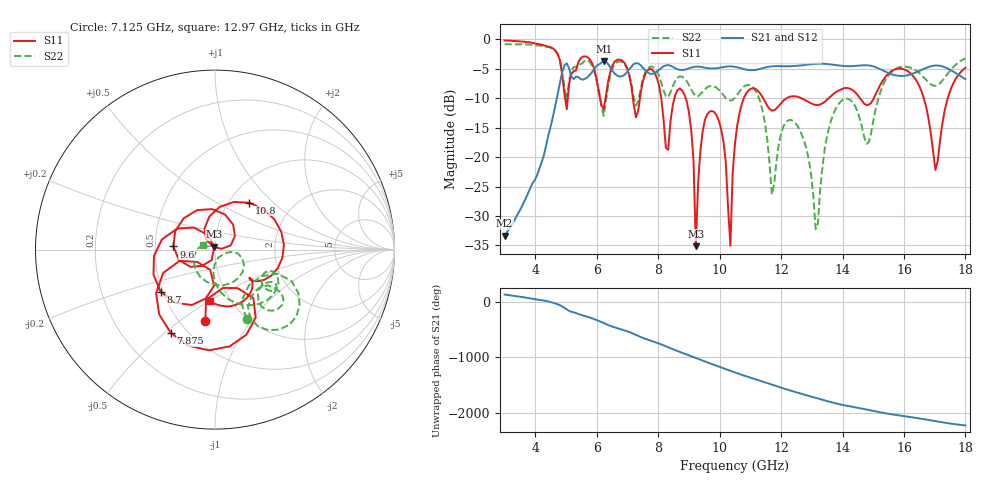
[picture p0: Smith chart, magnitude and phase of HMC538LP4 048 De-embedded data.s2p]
! Chelmsford, MA 01824
! http://www.hittite.com
! Tel: 978-250-3343
! Fax: 978-250-3373
! Device  :  HMC538LP4
! Description:  600 Analog Phase Shifter
! Frequency  :  6.0 GHz - 15.0 GHz
! Package  :  LP4  - 4x4 mm Quad Flatpack No-Lead (QFN) Plastic Package: 24 pin
! Ports  :  2 RF, 1 DC
!  Pin  3  = Rfin  = Port 1
!  Pin  16  = Rfout = Port 2
!  pin  21  = vCTL
! Voltages:  VCTL  = 0 to 5.0 Volts
! Currents :  Vb(V)  Vd(V)  Ib(mA)  Id(mA)
!  0.00  4.80  0.000000	0.483526
! Data:  The device was measured on evaluation board 111296-1.
!  Data was collected using a calibrated network analyzer.
!  The evaluation circuit board was modeled and simulated.This was use
!  to removed the evaluation board circuit from the measured data.
!  The reference plane is the center of the package pin.
! Misc:  Lot #
!Date Measured:  03 - 11 -2009
! Date:  03 - 17 -2009
! Note:
!  Hittite Microwave supplies this data as a sample of measured data at the
!  package pin for this package product.  Your particular data for this product
!  may vary.
!  Data was taken at 25 degrees C.
!  Hittite Microwave reserves the right to change this data at anytime.
# MHz S MA R 50
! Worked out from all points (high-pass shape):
!   201 points, 3 GHz to 18 GHz, reference 50 ohm
!   highest |S21| = -3.68 dB at 6.225 GHz (marker M1); lowest = -33.4 dB at 3 GHz (marker M2)
!   |S21| within 3 dB of the highest: 4.829 GHz to 5.239 GHz (410 MHz wide, 8.14 % of centre); 5.619 GHz to 17.98 GHz (12.36 GHz wide, 105 % of centre)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
!   lowest |S11| = -35.1 dB at 9.225 GHz (marker M3), VSWR 1.04, Z = 49.5 + j1.68 ohm
!   |S11| at or under -10 dB: 8.896 GHz to 10.79 GHz (1.891 GHz wide, 19.2 % of centre); 12.67 GHz to 13.55 GHz (881 MHz wide, 6.72 % of centre); 16.65 GHz to 17.43 GHz (779.4 MHz wide, 4.58 % of centre)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
!   |S22| runs from -32.2 to -0.8 dB; largest |S21 - S12| = 0.0021
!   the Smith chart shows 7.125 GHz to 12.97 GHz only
!   S11 on the Smith chart (normalised r, x): 7.125 GHz: 0.66, -0.63; 7.875 GHz: 0.41, -0.53; 8.7 GHz: 0.49, -0.27; 9.6 GHz: 0.62, +0.02; 10.8 GHz: 1.24, +0.72; 12.97 GHz: 0.81, -0.50
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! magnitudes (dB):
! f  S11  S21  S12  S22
! 3 GHz  -0.2  -33.4  -33.4  -0.8
! 5.55 GHz  -2.9  -6.8  -6.9  -4.0
! 6.225 GHz  -11.9  -3.7  -3.7  -13.0
! 7.125 GHz  -7.9  -4.6  -4.6  -7.5
! 7.875 GHz  -5.6  -5.7  -5.8  -4.9
! 8.025 GHz  -7.8  -5.2  -5.2  -6.2
! 8.325 GHz  -18.7  -4.4  -4.4  -9.8
! 8.7 GHz  -8.3  -5.2  -5.2  -6.3
! 9.075 GHz  -15.4  -4.8  -4.8  -8.5
! 9.225 GHz  -35.1  -4.6  -4.6  -9.6
! 9.6 GHz  -12.7  -4.9  -4.9  -8.1
! 10.12 GHz  -17.4  -4.7  -4.7  -9.5
! 10.35 GHz  -35.1  -4.6  -4.6  -10.4
! 10.5 GHz  -17.6  -4.7  -4.7  -9.9
! 10.8 GHz  -9.8  -5.1  -5.1  -8.0
! 11.7 GHz  -12.1  -4.6  -4.6  -26.3
! 12.22 GHz  -9.9  -4.6  -4.6  -13.8
! 12.97 GHz  -10.9  -4.2  -4.2  -22.8
! 13.05 GHz  -11.0  -4.2  -4.2  -26.6
! 15.53 GHz  -5.6  -5.8  -5.8  -5.9
! 17.02 GHz  -22.2  -4.4  -4.5  -7.9
! 18 GHz  -4.8  -6.7  -6.8  -3.2
